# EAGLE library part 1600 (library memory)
MEMORY
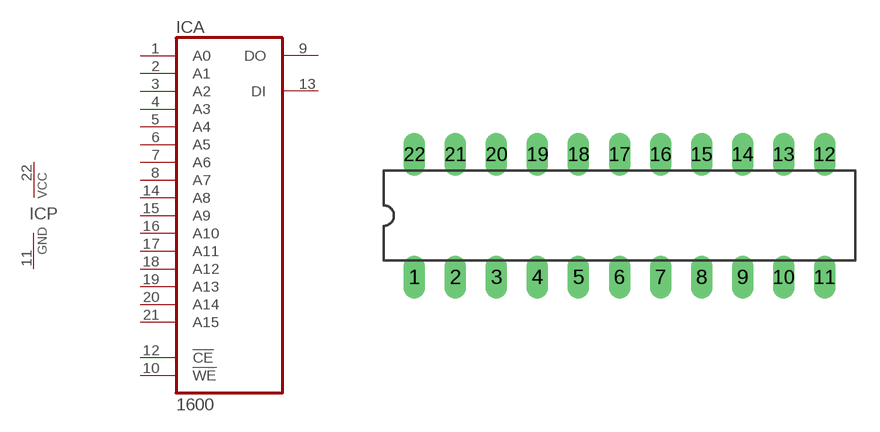
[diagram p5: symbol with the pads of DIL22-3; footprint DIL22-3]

Designator prefix IC; gates A=1600 P=PWRN

## 1600  [DIL22-3]
1  A:A0  in
2  A:A1  in
3  A:A2  in
4  A:A3  in
5  A:A4  in
6  A:A5  in
7  A:A6  in
8  A:A7  in
9  A:DO  hiz
10  A:!WE  in
11  P:GND  pwr
12  A:!CE  in
13  A:DI  in
14  A:A8  in
15  A:A9  in
16  A:A10  in
17  A:A11  in
18  A:A12  in
19  A:A13  in
20  A:A14  in
21  A:A15  in
22  P:VCC  pwr

## Footprint DIL22-3 (pad centres in mm)
Dual In Line Package 0.3 inch
drill 0.813 long: 1 -12.7,-3.81; 2 -10.16,-3.81; 3 -7.62,-3.81; 4 -5.08,-3.81; 5 -2.54,-3.81; 6 0,-3.81; 7 2.54,-3.81; 8 5.08,-3.81; 9 7.62,-3.81; 10 10.16,-3.81; 11 12.7,-3.81; 12 12.7,3.81; 13 10.16,3.81; 14 7.62,3.81; 15 5.08,3.81; 16 2.54,3.81; 17 0,3.81; 18 -2.54,3.81; 19 -5.08,3.81; 20 -7.62,3.81; 21 -10.16,3.81; 22 -12.7,3.81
